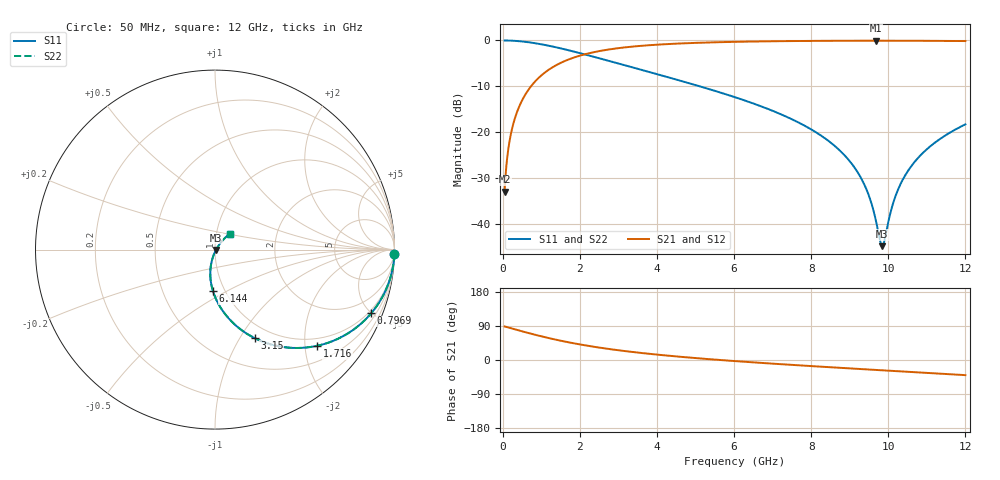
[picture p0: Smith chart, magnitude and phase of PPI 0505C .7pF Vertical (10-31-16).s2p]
# GHz S MA R 50
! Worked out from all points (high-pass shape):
!   1601 points, 50 MHz to 12 GHz, reference 50 ohm
!   highest |S21| = -0.06 dB at 9.685 GHz (marker M1); lowest = -32.9 dB at 50 MHz (marker M2)
!   |S21| within 3 dB of the highest: 2.11 GHz to end of sweep
!   lowest |S11| = -44.7 dB at 9.842 GHz (marker M3), VSWR 1.01, Z = 50.5 - j0.282 ohm
!   |S11| at or under -10 dB: 5.121 GHz to end of sweep
!   |S22| runs from -44.7 to 0.0 dB; largest |S21 - S12| = 0
!   S11 on the Smith chart (normalised r, x): 50 MHz: 1, -79; 796.9 MHz: 0.82, -4.96; 1.716 GHz: 0.82, -2.26; 3.15 GHz: 0.83, -1.16; 6.144 GHz: 0.88, -0.43; 12 GHz: 1.16, +0.21
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0.05  0.9997 -1.4  0.02268 88.6  0.02268 88.6  0.9997 -1.4
0.1695  0.997 -4.9  0.07671 85.1  0.07671 85.1  0.997 -4.9
0.3039375  0.9906 -8.7  0.1367 81.3  0.1367 81.3  0.9906 -8.7
0.5130625  0.9737 -14.6  0.2272 75.4  0.2272 75.4  0.9737 -14.6
0.796875  0.9396 -22.2  0.3415 67.7  0.3415 67.7  0.9396 -22.2
1.715531  0.7812 -43.4  0.6226 46.5  0.6226 46.5  0.7812 -43.4
2.044156  0.7206 -49.5  0.6913 40.3  0.6913 40.3  0.7206 -49.5
3.149531  0.54 -65.9  0.8388 23.8  0.8388 23.8  0.54 -65.9
4.038312  0.4259 -75.7  0.9013 13.9  0.9013 13.9  0.4259 -75.7
6.025  0.2414 -91.9  0.9659 -2.9  0.9659 -2.9  0.2414 -91.9
6.1445  0.2324 -92.7  0.9681 -3.7  0.9681 -3.7  0.2324 -92.7
8.019156  0.1067 -103.5  0.9888 -16.2  0.9888 -16.2  0.1067 -103.5
8.654  0.06876 -105.7  0.9918 -20.1  0.9918 -20.1  0.06876 -105.7
9.124531  0.04151 -105.4  0.9931 -22.9  0.9931 -22.9  0.04151 -105.4
9.453156  0.02297 -100.7  0.9935 -24.9  0.9935 -24.9  0.02297 -100.7
9.684688  0.01073 -84.0  0.9936 -26.3  0.9936 -26.3  0.01073 -84.0
9.841531  0.005794 -28.9  0.9936 -27.2  0.9936 -27.2  0.005794 -28.9
10.01331  0.01122 30.2  0.9934 -28.2  0.9934 -28.2  0.01122 30.2
10.27472  0.02506 46.4  0.9931 -29.8  0.9931 -29.8  0.02506 46.4
10.66309  0.04666 50.3  0.9921 -32.0  0.9921 -32.0  0.04666 50.3
11.23819  0.07902 49.9  0.9897 -35.4  0.9897 -35.4  0.07902 49.9
12  0.1224 46.9  0.9849 -39.9  0.9849 -39.9  0.1224 46.9
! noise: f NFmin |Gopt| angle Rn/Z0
0.05  0.001452  0.9778  1.245  0.01491
1.372  0.005849  0.7746  6.982  0.005283
2.701  0.009141  0.718  10.09  0.006363
4.031  0.01207  0.6854  13.31  0.007349
5.36  0.01483  0.6638  16.55  0.008285
6.682  0.01752  0.649  19.74  0.009213
8.012  0.02024  0.6391  22.92  0.01018
9.341  0.02301  0.6331  26.04  0.01122
10.67  0.0259  0.6305  29.11  0.01237
12  0.02895  0.6308  32.13  0.01365
